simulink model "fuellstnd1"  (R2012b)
settings: Solver=ode45  StartTime=0.0  StopTime=10.0  RelTol=1e-3
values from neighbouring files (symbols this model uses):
  A1 = 0.02    [fuellstnd_1.m]    (also in fuellstnd_2.m; fuellstnd_21.m; fuellstnd_3.m; fuellstnd_31.m)
  A12 = 0.005    [fuellstnd_1.m]    (also in fuellstnd_2.m; fuellstnd_21.m; fuellstnd_3.m; fuellstnd_31.m)
  A2 = A1    (= 0.02)    [fuellstnd_1.m]    (also in fuellstnd_2.m; fuellstnd_21.m; fuellstnd_3.m; fuellstnd_31.m)
  A23 = A12    (= 0.005)    [fuellstnd_1.m]    (also in fuellstnd_2.m; fuellstnd_21.m; fuellstnd_3.m; fuellstnd_31.m)
  A3 = A1    (= 0.02)    [fuellstnd_1.m]    (also in fuellstnd_2.m; fuellstnd_21.m; fuellstnd_3.m; fuellstnd_31.m)
  A30 = A12    (= 0.005)    [fuellstnd_1.m]    (also in fuellstnd_2.m; fuellstnd_21.m; fuellstnd_3.m; fuellstnd_31.m)
  g = 9.89    [fuellstnd_1.m]    (also in fuellstnd_2.m; fuellstnd_21.m; fuellstnd_3.m; fuellstnd_31.m)
  h10 = 0.0    (= 0)    [fuellstnd_1.m]    (also in fuellstnd_2.m; fuellstnd_21.m; fuellstnd_3.m; fuellstnd_31.m)
  h20 = h10    (= 0)    [fuellstnd_1.m]    (also in fuellstnd_2.m; fuellstnd_21.m; fuellstnd_3.m; fuellstnd_31.m)
  h30 = h10    (= 0)    [fuellstnd_1.m]    (also in fuellstnd_2.m; fuellstnd_21.m; fuellstnd_3.m; fuellstnd_31.m)
  Qz = 0.005,    [fuellstnd_1.m]    (also in fuellstnd_3.m = 0.05,; fuellstnd_31.m = 0.05,; linear_fuellstnd_1.m)
  Qz1 = 0.01,    [fuellstnd_1.m]

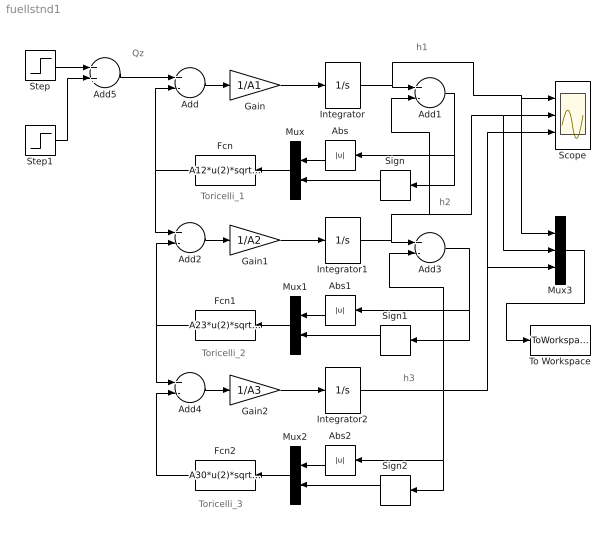
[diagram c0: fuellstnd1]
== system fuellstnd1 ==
  note: h3
  note: h2
  note: h1
  note: Toricelli_3
  note: Toricelli_2
  note: Toricelli_1
  note: Qz
  Abs : Abs
  Abs1 : Abs
  Abs2 : Abs
  Add{,1..4} (5 alike) : Sum  Inputs=+-
  Add5 : Sum
  Fcn : Fcn  Expr=A12*u(2)*sqrt(2*g*u(1))
  Fcn1 : Fcn  Expr=A23*u(2)*sqrt(2*g*u(1))
  Fcn2 : Fcn  Expr=A30*u(2)*sqrt(2*g*u(1))
  Gain : Gain  Gain=1/A1
  Gain1 : Gain  Gain=1/A2
  Gain2 : Gain  Gain=1/A3
  Integrator : Integrator  InitialCondition=h10
  Integrator1 : Integrator  InitialCondition=h20
  Integrator2 : Integrator  InitialCondition=h30
  Mux : Mux  Inputs=2
  Mux1 : Mux  Inputs=2
  Mux2 : Mux  Inputs=2
  Mux3 : Mux  Inputs=3
  Scope : Scope  NumInputPorts=3
  Sign : Signum
  Sign1 : Signum
  Sign2 : Signum
  Step : Step  Time=0  After=Qz1  SampleTime=0
  Step1 : Step  Time=100  After=Qz  SampleTime=0  ZeroCross=off
  To Workspace : ToWorkspace  VariableName=y  SampleTime=-1  SaveFormat=Structure With Time
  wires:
  Add/1 -> Gain/1
  Gain/1 -> Integrator/1
  Add1/1 -> Sign/1, Abs/1
  Abs/1 -> Mux/1
  Sign/1 -> Mux/2
  Mux/1 -> Fcn/1
  Fcn/1 -> Add/2, Add2/1
  Add2/1 -> Gain1/1
  Gain1/1 -> Integrator1/1
  Abs1/1 -> Mux1/1
  Sign1/1 -> Mux1/2
  Mux1/1 -> Fcn1/1
  Fcn1/1 -> Add4/1, Add2/2
  Add4/1 -> Gain2/1
  Gain2/1 -> Integrator2/1
  Abs2/1 -> Mux2/1
  Sign2/1 -> Mux2/2
  Mux2/1 -> Fcn2/1
  Fcn2/1 -> Add4/2
  Integrator2/1 -> Mux3/3, Scope/3, Sign2/1, Abs2/1, Add3/2
  Add3/1 -> Abs1/1, Sign1/1
  Mux3/1 -> To Workspace/1
  Add5/1 -> Add/1
  Step/1 -> Add5/1
  Step1/1 -> Add5/2
  Integrator1/1 -> Mux3/2, Scope/2, Add1/2, Add3/1
  Integrator/1 -> Mux3/1, Scope/1, Add1/1
